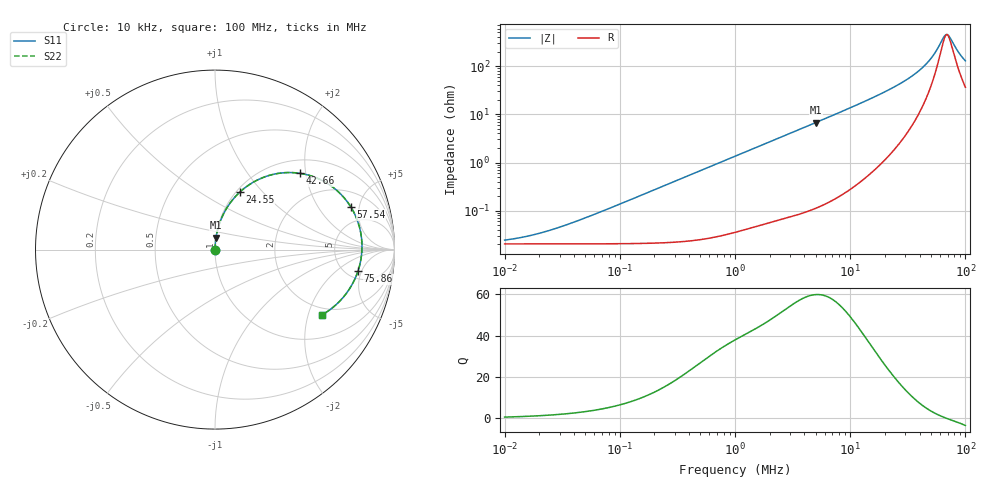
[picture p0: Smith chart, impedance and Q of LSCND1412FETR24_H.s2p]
! LSCND1412FETR24_H  S-PARAMETER MODEL  ( Standard Model )
! Model Generated by TAIYO YUDEN Corporation (http://www.ty-top.com)
! Version 1.0
! TAIYO YUDEN Control No. 241002
! Copyright(c) 2024 TAIYO YUDEN CO.,LTD. All Rights Reserved.
! Product Description (link to TY-COMPAS)
! https://ds.yuden.co.jp/TYCOMPAS/or/detail?pn=LSCND1412FETR24MH&u=M
! Products Name : Inductors
! Characteristics :
!  Inductance : 0.24 [uH] , SRF(min) : - [Hz] , DC Resistance(max) : 23 [mOhm]
!  Rated Current : Saturation  6.6 [A] (dL = 30 [%]), Temp Rise  4.2 [A] (dT = 40 [degC])
!  Case Size : 1.4 x 1.2 / 0.055 x 0.047 [mm/inch] , Thickness : 0.65 / 0.026 [mm/inch]
!  (Conditions: Temperature = 25 [degC] , DC Bias Current = 0 [A])
! External Node Assignments :
!  1  o---GGG---o  2
! GND o---------o GND
! Frequency Range : 10kHz  -  100MHz  [ 402 STEP ]
# MHz S RI R 50
! Freq[MHz].  S11 Real  S11 Imag  S21 Real  S21 Imag  S12 Real  S12 Imag  S22 Real  S22 Imag
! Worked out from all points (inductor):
!   401 points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, 10 kHz to 100 MHz, reference 50 ohm
!   read as one part in series: L = 216 nH near 45.71 kHz
!   highest Q = 59.8 at 5.012 MHz (marker M1), where L = 213 nH
!   self-resonance near 69.13 MHz
!   S11 on the Smith chart (normalised r, x): 10 kHz: 1.00, +0.00; 24.55 MHz: 1.04, +0.75; 42.66 MHz: 1.30, +1.85; 57.54 MHz: 3.21, +4.12; 75.86 MHz: 6.28, -4.31; 100 MHz: 1.73, -2.45
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0.01  0.000205 0.000136  0.9998 -0.000136  0.9998 -0.000136  0.000205 0.000136
0.014125  0.000205 0.000192  0.9998 -0.000192  0.9998 -0.000192  0.000205 0.000192
0.020417  0.000205 0.000277  0.9998 -0.000277  0.9998 -0.000277  0.000205 0.000277
0.046774  0.000206 0.000635  0.9998 -0.000635  0.9998 -0.000635  0.000206 0.000635
0.218776  0.000223 0.00297  0.9998 -0.00297  0.9998 -0.00297  0.000223 0.00297
1  0.000537 0.0135  0.9995 -0.0135  0.9995 -0.0135  0.000537 0.0135
4.677351  0.00494 0.0622  0.9951 -0.0622  0.9951 -0.0622  0.00494 0.0622
5.011872  0.00559 0.0666  0.9944 -0.0666  0.9944 -0.0666  0.00559 0.0666
11.22019  0.0262 0.149  0.9738 -0.149  0.9738 -0.149  0.0262 0.149
16.2181  0.0558 0.2148  0.9442 -0.2148  0.9442 -0.2148  0.0558 0.2148
21.87762  0.1062 0.2871  0.8938 -0.2871  0.8938 -0.2871  0.1062 0.2871
24.54709  0.1371 0.3192  0.8629 -0.3192  0.8629 -0.3192  0.1371 0.3192
33.11311  0.2705 0.4027  0.7295 -0.4027  0.7295 -0.4027  0.2705 0.4027
42.65795  0.4728 0.4251  0.5272 -0.4251  0.5272 -0.4251  0.4728 0.4251
50.11872  0.6358 0.3627  0.3642 -0.3627  0.3642 -0.3627  0.6358 0.3627
57.54399  0.7571 0.2372  0.2429 -0.2372  0.2429 -0.2372  0.7571 0.2372
64.56542  0.8123 0.0924  0.1877 -0.0924  0.1877 -0.0924  0.8123 0.0924
67.6083  0.8188 0.0301  0.1812 -0.0301  0.1812 -0.0301  0.8188 0.0301
70.79458  0.8162 -0.0318  0.1838 0.0318  0.1838 0.0318  0.8162 -0.0318
75.85776  0.7965 -0.1205  0.2035 0.1205  0.2035 0.1205  0.7965 -0.1205
87.09636  0.7125 -0.2682  0.2875 0.2682  0.2875 0.2682  0.7125 -0.2682
100  0.5943 -0.3646  0.4057 0.3646  0.4057 0.3646  0.5943 -0.3646
